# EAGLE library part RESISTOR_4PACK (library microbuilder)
Resistor Packs (4 resistors) 4 x 0603 10K 1/16W - Digikey: YC164J-10KCT-ND
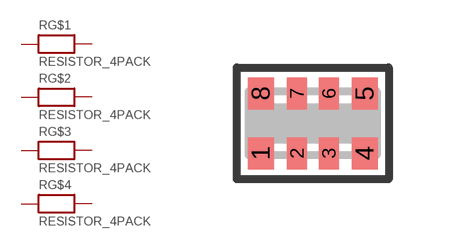
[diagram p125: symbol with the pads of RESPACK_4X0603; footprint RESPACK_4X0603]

Designator prefix R; gates G$1=RESISTOR G$2=RESISTOR G$3=RESISTOR G$4=RESISTOR

## RESISTOR_4PACK  [RESPACK_4X0603]
1  G$1:1  pas
2  G$2:1  pas
3  G$3:1  pas
4  G$4:1  pas
5  G$4:2  pas
6  G$3:2  pas
7  G$2:2  pas
8  G$1:2  pas

## Footprint RESPACK_4X0603 (pad centres in mm)
smd 0.65 x 0.8: 1 -1.3,-0.75; 4 1.3,-0.75; 5 1.3,0.75; 8 -1.3,0.75
smd 0.5 x 0.8: 2 -0.4,-0.75; 3 0.4,-0.75; 6 0.4,0.75; 7 -0.4,0.75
